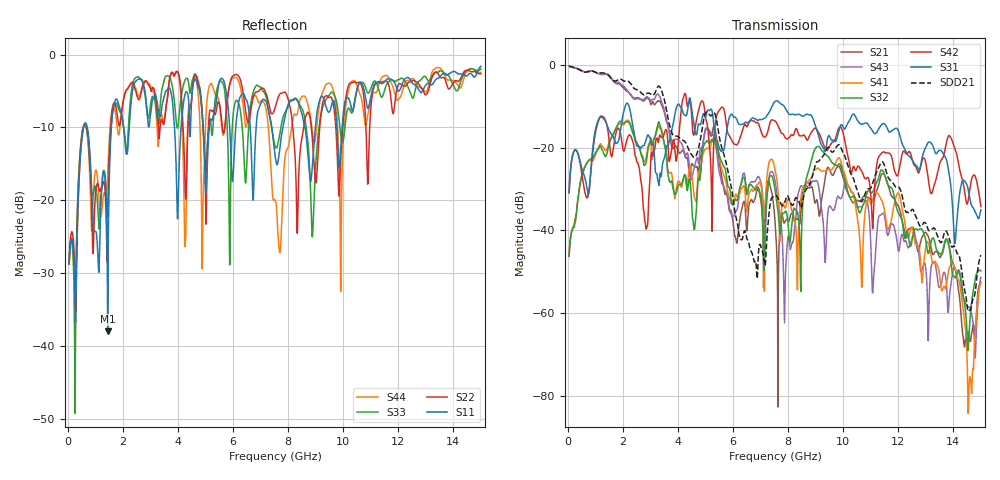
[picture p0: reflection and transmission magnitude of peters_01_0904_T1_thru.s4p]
# MHZ S RI R 50.00
! FREQ  S11  S12  S13  S14
!  S21  S22  S23  S24
!  S31  S32  S33  S34
!  S41  S42  S43  S44
!  REAL  IMAG  REAL  IMAG  REAL  IMAG  REAL  IMAG
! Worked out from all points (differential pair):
!   1496 points, 50 MHz to 15 GHz, reference 50 ohm
!   strongest paths, dB at 50 MHz, 3.79 GHz, 7.53 GHz, 11.27 GHz, 15 GHz:
!     S31: -30.9, -15.3, -8.8, -15.7, -35.0
!     S42: -30.9, -19.8, -13.5, -22.5, -34.2
!     S32: -46.3, -28.6, -30.3, -27.6, -49.8
!     S41: -46.2, -26.9, -25.4, -31.1, -52.8
!     S43: -0.2, -18.4, -28.1, -37.4, -51.4
!     S21: -0.2, -20.1, -38.3, -29.4, -52.5
!   taken as a pair (ports 3,1 in; 4,2 out), SDD21 dB: -0.2, -16.5, -31.6, -25.0, -46.0
!   lowest |S11| = -38.0 dB at 1.45 GHz (marker M1), VSWR 1.03, Z = 49.7 - j1.22 ohm
!   |S11| at or under -10 dB: start of sweep to 575 MHz; 702.7 MHz to 1.583 GHz (880.3 MHz wide, 77 % of centre); 7.41 GHz to 7.812 GHz (402.5 MHz wide, 5.29 % of centre)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
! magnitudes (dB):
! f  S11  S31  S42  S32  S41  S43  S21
! 50 MHz  -28.8  -30.9  -30.9  -46.3  -46.2  -0.2  -0.2
! 1.45 GHz  -38.0  -14.9  -15.5  -20.6  -19.9  -2.3  -2.2
! 2.85 GHz  -6.6  -18.0  -39.7  -23.4  -22.3  -7.7  -8.1
! 7.88 GHz  -8.7  -10.2  -17.4  -35.6  -34.5  -58.4  -38.0
! 12.01 GHz  -5.0  -16.0  -26.0  -35.9  -31.0  -45.0  -34.2
! 14.59 GHz  -2.6  -31.9  -30.3  -62.9  -75.4  -58.6  -66.4
! 15 GHz  -1.6  -35.0  -34.2  -49.8  -52.8  -51.4  -52.5
